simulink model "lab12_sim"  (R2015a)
settings: Solver=ode45  SolverMode=SingleTasking  StartTime=0.0  StopTime=10  RelTol=1e-3
undefined symbols (not defined in the file): C_pid
libraries: cstblocks x4

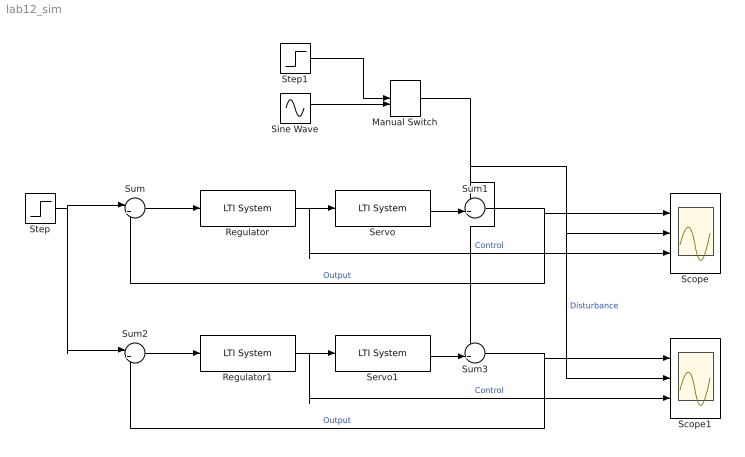
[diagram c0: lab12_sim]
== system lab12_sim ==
  Manual Switch : ManualSwitch  CurrentSetting=0
  Regulator : cstblocks/LTI System  sys=K  IC=[]
  Regulator1 : cstblocks/LTI System  sys=tf(C_pid)  IC=[]
  Scope : Scope  NumInputPorts=3
  Scope1 : Scope  NumInputPorts=3
  Servo : cstblocks/LTI System  sys=G_rand  IC=[]
  Servo1 : cstblocks/LTI System  sys=G_rand  IC=[]
  Sine Wave : Sin  Amplitude=0.1  Frequency=2  SampleTime=0
  Step : Step  SampleTime=0
  Step1 : Step  Time=3  After=.1  SampleTime=0
  Sum : Sum  Inputs=|+-
  Sum1 : Sum  Inputs=++|
  Sum2 : Sum  Inputs=|+-
  Sum3 : Sum  Inputs=++|
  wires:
  Regulator/1 -> Scope/3, Servo/1  "Control"
  Sum/1 -> Regulator/1
  Sum1/1 -> Scope/1, Sum/2  "Output"
  Servo/1 -> Sum1/2
  Step1/1 -> Manual Switch/1
  Sine Wave/1 -> Manual Switch/2
  Manual Switch/1 -> Sum3/1, Sum1/1, Scope1/2, Scope/2  "Disturbance"
  Servo1/1 -> Sum3/2
  Sum3/1 -> Scope1/1, Sum2/2  "Output"
  Step/1 -> Sum2/1, Sum/1
  Regulator1/1 -> Scope1/3, Servo1/1  "Control"
  Sum2/1 -> Regulator1/1
